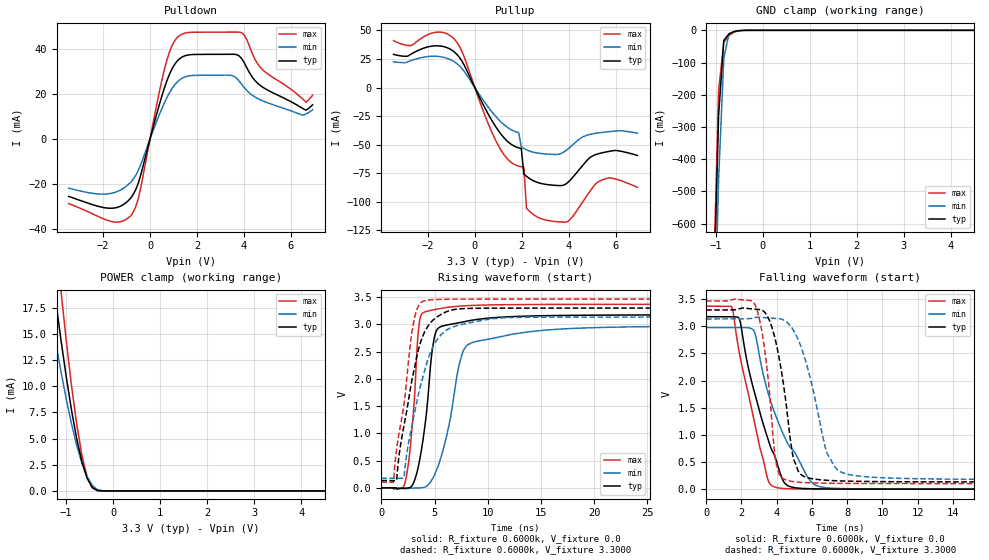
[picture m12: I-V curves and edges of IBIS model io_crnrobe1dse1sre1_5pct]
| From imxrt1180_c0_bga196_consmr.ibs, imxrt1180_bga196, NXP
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[Model]  io_crnrobe1dse1sre1_5pct
|   Model io_crnrobe1dse1sre1_5pct
| This model was characterised for following simulation conditions:
| External (pad) voltage:
|   - Typ: 3.3V,   - Min: 3.135V,   - Max: 3.465V
| Library cells for typ/min/max conditions are connected as defined below:
|  PAD_IO - External Pad
|  ipp_do - Core Input
|  ipp_obe - Output Buffer Enable
|  ASRCN3V3[3] - NC
|  ASRCN3V3[4] - NC
|  ASRCP3V3[4] - NC
|  REFAPBIAS3V3 - gnde
|  REFBAMPL3V3 - vdd1v8
|  REFCAMPH3V3 - vdd1v8
|  REFDNBIAS3V3 - vdd1v8
|  REFH3V3 - REFH3V3
|  REFL3V3 - REFL3V3
|  gnde - gnde
|  ipp_dse - vdd
|  ipp_ina235_3v - NC
|  ipp_ina40_3v - NC
|  ipp_ina_mux - NC
|  ipp_ind - NC
|  ipp_ind_1p8v - NC
|  ipp_ind_3v - NC
|  ipp_sre - vdd
|  vdd - vdd
|  vdd1v8 - vdd1v8
|  vdda - vdde3v3
|  vdde3v3 - vdde3v3
| All other pins connected to ground
Model_type I/O
Polarity   Non-Inverting
Enable   Active-High
Vinl =   0.9900V
Vinh =   2.3100V
Vmeas =  1.6500V
Cref =   15.0000pF
Rref =   0.6000k
Vref =   0.0V
C_comp   4.0038pF   3.8208pF   4.1241pF
|C_comp_pullup   0.5150pF   0.5903pF   0.4959pF
|C_comp_pulldown   2.0814pF   2.1809pF   1.8612pF
[Model Spec]
| variable   typ   min   max
Vinh   2.3100V   NA   NA
Vinl   0.9900V   NA   NA
Vref   0.0V   0.0V   0.0V
Cref   15.0000pF   15.0000pF   15.0000pF
Rref   0.6000k   0.6000k   0.6000k
[Receiver Thresholds]
Vcross_high  =   0.0V
Vcross_low  =   0.0V
Vdiff_ac  =   0.0V
Vdiff_dc  =   0.0V
Tdiffslew_ac  =   0.0S
[Temperature Range]   25.0000   0.1250k   -40.0000
[Voltage Range]   3.3000V   3.1350V   3.4650V
[Pullup Reference]   3.3000V   3.1350V   3.4650V
[Pulldown Reference]   0.0V   0.0V   0.0V
[POWER Clamp Reference]   3.3000V   3.1350V   3.4650V
[GND Clamp Reference]   0.0V   0.0V   0.0V
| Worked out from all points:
|   slope of the pulldown table from 0 to 0.495 V, typ, clamps not added: 26.4 ohm
|   slope of the pullup table from 0 to 0.495 V, typ, clamps not added: 24.4 ohm
|   GND clamp passes 1 mA (typ) near -0.50 V on its own axis
|   POWER clamp passes 1 mA (typ) near -0.52 V on its own axis
|   rising waveform, R_fixture 0.6000k, V_fixture 0.0: 20-80 % time 1.08ns typ, 1.82ns min, 718ps max; typ from 0 V to 3.18 V
|   rising waveform, R_fixture 0.6000k, V_fixture 3.3000: 20-80 % time 1.89ns typ, 2.24ns min, 1.34ns max; typ from 0.133 V to 3.3 V
|   falling waveform, R_fixture 0.6000k, V_fixture 0.0: 20-80 % time 1.65ns typ, 2.1ns min, 1.34ns max; typ from 3.18 V to 0 V
|   falling waveform, R_fixture 0.6000k, V_fixture 3.3000: 20-80 % time 855ps typ, 1.29ns min, 633ps max; typ from 3.3 V to 0.133 V
[Pulldown]
|Voltage   I(typ)   I(min)   I(max)
-3.465V   -25.47mA   -21.79mA   -28.66mA
-1.595V   -30.68mA   -23.95mA   -36.7mA
-715mV    -24.55mA   -17.79mA   -32.46mA
-495mV    -19.43mA   -13.83mA   -26.26mA
715mV     25.71mA    18.31mA    34.82mA
1.045V    33.06mA    23.94mA    43.49mA
1.375V    36.41mA    26.97mA    46.59mA
3.465V    37.59mA    28.21mA    47.43mA
3.905V    35.69mA    24.29mA    47.16mA
4.895V    22.39mA    16.52mA    29.84mA
6.655V    12.8mA     11.14mA    16.38mA
6.93V     15.19mA    12.98mA    19.44mA
[Pullup]
|Voltage   I(typ)   I(min)   I(max)
-3.465V   29.1mA     22.59mA    41.21mA
-1.54V    36.55mA    27.24mA    48.59mA
-770mV    29.19mA    21.06mA    39.85mA
990mV     -37.26mA   -27.44mA   -50.23mA
1.87V     -52.73mA   -39.38mA   -68.73mA
1.98V     -53.28mA   -51.96mA   -69.28mA
2.09V     -75.64mA   -53.32mA   -69.65mA
2.2V      -77.6mA    -54.45mA   -105.5mA
2.64V     -82.78mA   -57.16mA   -113mA
3.96V     -83.1mA    -53.87mA   -117.2mA
5.61V     -56.28mA   -38.79mA   -79.56mA
6.93V     -59.4mA    -39.92mA   -87.28mA
[GND_clamp]
|Voltage   I(typ)   I(min)   I(max)
-3.465V   -18.65A    -18.54A    -19.59A
-1.045V   -856.3mA   -1.07A     -789.2mA
-935mV    -262.9mA   -462.2mA   -186.4mA
-825mV    -31.14mA   -87.01mA   -37.16mA
-715mV    -11.21mA   -10.51mA   -15.88mA
-605mV    -3.859mA   -3.519mA   -5.394mA
-385mV    -79.67uA   -219.6uA   -43.93uA
6.93V     0A         0A         0A
[POWER_clamp]
|Voltage   I(typ)   I(min)   I(max)
-3.465V   98.91mA    78.43mA    126mA
-1.43V    25.78mA    19.9mA     34.19mA
-1.32V    21.78mA    16.89mA    28.92mA
-1.21V    17.92mA    14mA       23.79mA
-1.1V     14.24mA    11.26mA    18.86mA
-880mV    7.673mA    6.373mA    9.998mA
-770mV    4.965mA    4.333mA    6.33mA
-660mV    2.777mA    2.644mA    3.379mA
-550mV    1.212mA    1.363mA    1.332mA
-440mV    333.5uA    531.5uA    282.6uA
-330mV    37.61uA    130.9uA    15.04uA
6.93V     0A         0A         0A
[Ramp]
| variable   typ   min   max
dV/dt_r  1.9062/1.0759n   1.7862/1.8175n   2.0217/0.7178n
dV/dt_f  1.9001/0.8555n   1.7755/1.2926n   2.0172/0.6326n
R_load = 0.6000k
[Rising Waveform]
R_fixture= 0.6000k
V_fixture= 0.0
V_fixture_min= 0.0
V_fixture_max= 0.0
|time   V(typ)   V(min)   V(max)
0s        57.42nV    1.437uV    26.77nV
2.232ns   -7.474mV   -19.35mV   98.69mV
2.851ns   28.4mV     -6.886mV   1.006V
3.553ns   459.1mV    -2.814mV   3.002V
4.296ns   1.473V     35.66mV    3.24V
4.746ns   2.47V      143.1mV    3.262V
5.193ns   2.891V     324mV      3.278V
7.529ns   3.039V     2.414V     3.338V
8.745ns   3.084V     2.678V     3.35V
60ns      3.177V     2.977V     3.369V
[Rising Waveform]
R_fixture= 0.6000k
V_fixture= 3.3000
V_fixture_min= 3.1350
V_fixture_max= 3.4650
|time   V(typ)   V(min)   V(max)
0s        133.2mV    175.8mV    103mV
1.133ns   132.5mV    175.8mV    100mV
1.431ns   138.4mV    175.5mV    703mV
2.114ns   1.125V     179.4mV    1.516V
3.035ns   2.122V     1.282V     3.042V
3.978ns   2.822V     2.087V     3.431V
4.787ns   3.066V     2.562V     3.454V
5.911ns   3.214V     2.865V     3.462V
10.42ns   3.298V     3.103V     3.465V
60ns      3.3V       3.135V     3.465V
[Falling Waveform]
R_fixture= 0.6000k
V_fixture= 0.0
V_fixture_min= 0.0
V_fixture_max= 0.0
|time   V(typ)   V(min)   V(max)
0s        3.177V     2.978V     3.369V
1.429ns   3.178V     2.978V     3.361V
1.871ns   3.14V      2.977V     2.53V
2.746ns   1.776V     2.89V      1.218V
3.519ns   909.6mV    1.764V     160.4mV
4.099ns   393.3mV    1.226V     22.63mV
4.596ns   71.19mV    860.3mV    8.148mV
5.881ns   8.115mV    163.2mV    1.323mV
7.048ns   2.996mV    20mV       372.9uV
60ns      1.076uV    2.051uV    865.4nV
[Falling Waveform]
R_fixture= 0.6000k
V_fixture= 3.3000
V_fixture_min= 3.1350
V_fixture_max= 3.4650
|time   V(typ)   V(min)   V(max)
0s        3.3V       3.135V     3.465V
2.806ns   3.315V     3.163V     3.371V
3.356ns   3.244V     3.158V     2.479V
3.962ns   2.699V     3.145V     486.6mV
4.337ns   2.038V     3.125V     199mV
4.828ns   793.9mV    2.987V     144.9mV
5.35ns    278.4mV    2.65V      125.6mV
6.891ns   162.2mV    637.6mV    109.1mV
8.357ns   145.6mV    253.7mV    105.2mV
60ns      133.2mV    175.8mV    103mV
